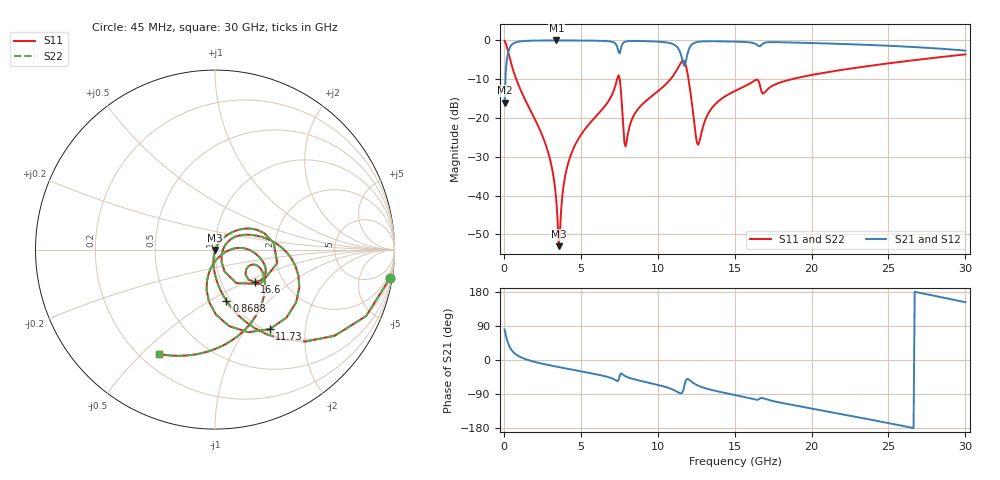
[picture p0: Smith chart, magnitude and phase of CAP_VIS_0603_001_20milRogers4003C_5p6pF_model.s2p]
! S-parameter model data by Modelithics Inc.  support@modelithics.com  813-866-6335  Tampa FL USA
! S-Parameter data specifications:
! Substrate: 20-mil Rogers 4003C, substrate thickness, H=0.508mm, Dielectric constant, Er=3.75
! PCB Mounting Pad Footprint: Pad width, PadW=0.90mm , Pad length, PadL=1.00mm , Pad gap, PadG (edge-to-edge)=1.00mm , Reference planes=3.0mm apart
! Created Wed Nov 18 13:23:57 2015
# hz S ma R 50
! 2 Port Network Data from SP1.SP block
! freq  magS11  angS11  magS21  angS21  magS12  angS12  magS22  angS22
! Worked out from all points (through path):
!   401 points, 45 MHz to 30 GHz, reference 50 ohm
!   highest |S21| = -0.02 dB at 3.415 GHz (marker M1); lowest = -16.0 dB at 45 MHz (marker M2)
!   group delay of S21, straight-line fit = 19.9 ps
!   lowest |S11| = -53.0 dB at 3.565 GHz (marker M3), VSWR 1.00, Z = 50.2 - j0.151 ohm
!   |S11| at or under -10 dB: 802.1 MHz to 7.361 GHz (6.559 GHz wide, 161 % of centre); 7.535 GHz to 10.83 GHz (3.294 GHz wide, 35.9 % of centre); 12 GHz to 18.71 GHz (6.711 GHz wide, 43.7 % of centre)
!   |S22| runs from -53.0 to -0.1 dB; largest |S21 - S12| = 0
!   S11 on the Smith chart (normalised r, x): 45 MHz: 1, -12; 868.8 MHz: 0.95, -0.59; 11.73 GHz: 1.04, -1.30; 16.6 GHz: 1.44, -0.57; 30 GHz: 0.27, -0.57
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4.5e7  0.9874 -9.3  0.1582 80.7  0.1582 80.7  0.9874 -9.3
3.4455e8  0.6283 -52.8  0.7774 37.1  0.7774 37.1  0.6283 -52.8
8.687625e8  0.2917 -77.4  0.9555 12.4  0.9555 12.4  0.2917 -77.4
2.815838e9  0.03946 -100.0  0.9972 -12.6  0.9972 -12.6  0.03946 -100.0
3.414938e9  0.008212 -93.5  0.9977 -17.6  0.9977 -17.6  0.008212 -93.5
3.564712e9  0.002236 -42.3  0.9976 -18.8  0.9976 -18.8  0.002236 -42.3
4.163812e9  0.02565 61.5  0.997 -23.4  0.997 -23.4  0.02565 61.5
5.062462e9  0.06302 57.2  0.9948 -30.3  0.9948 -30.3  0.06302 57.2
7.383975e9  0.3288 6.7  0.8046 -55.9  0.8046 -55.9  0.3288 6.7
7.983075e9  0.05097 13.2  0.9712 -44.6  0.9712 -44.6  0.05097 13.2
8.582175e9  0.12 33.1  0.9821 -52.1  0.9821 -52.1  0.12 33.1
1.007992e10  0.227 20.8  0.9615 -66.3  0.9615 -66.3  0.227 20.8
1.112835e10  0.382 0.3  0.8669 -80.9  0.8669 -80.9  0.382 0.3
1.172745e10  0.5375 -55.6  0.4685 -69.1  0.4685 -69.1  0.5375 -55.6
1.210189e10  0.2316 -101.6  0.8279 -54.0  0.8279 -54.0  0.2316 -101.6
1.26261e10  0.04524 -45.4  0.9568 -67.7  0.9568 -67.7  0.04524 -45.4
1.352475e10  0.1349 4.0  0.9738 -79.2  0.9738 -79.2  0.1349 4.0
1.50225e10  0.2232 -5.1  0.9631 -92.5  0.9631 -92.5  0.2232 -5.1
1.659514e10  0.2865 -39.3  0.8384 -103.1  0.8384 -103.1  0.2865 -39.3
2.003996e10  0.3594 -39.6  0.9241 -128.4  0.9241 -128.4  0.3594 -39.6
2.505742e10  0.5075 -77.7  0.8517 -167.0  0.8517 -167.0  0.5075 -77.7
3e10  0.66 -118.1  0.739 152.5  0.739 152.5  0.66 -118.1
